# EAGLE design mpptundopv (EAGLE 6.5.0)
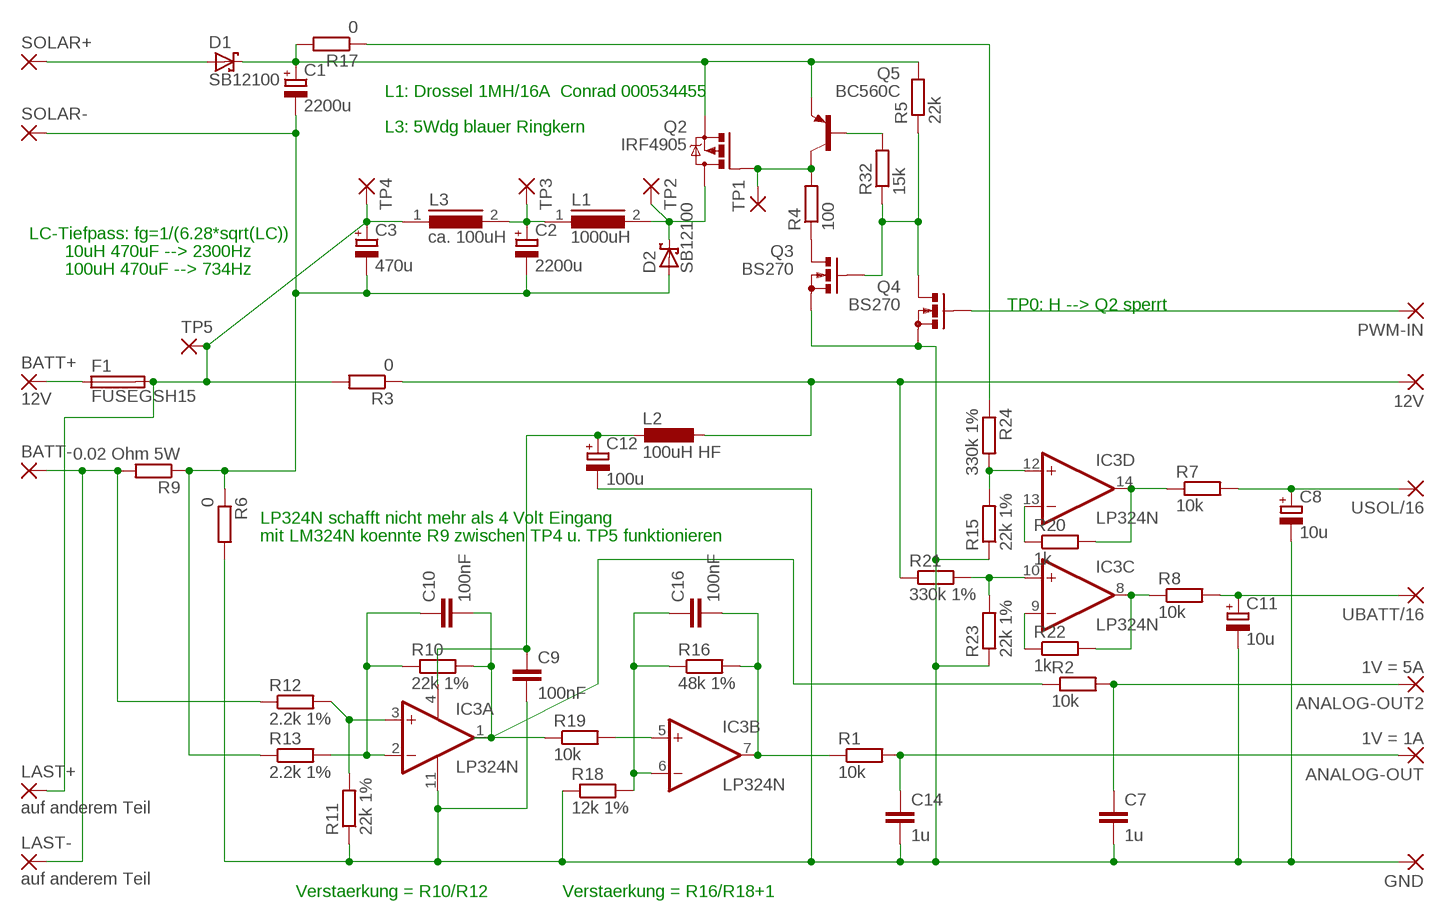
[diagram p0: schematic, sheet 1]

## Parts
12V  WIREPAD2,15/1,0  [2,15/1,0]
ANALOG-OUT  1V = 1A  WIREPAD2,15/1,0  [2,15/1,0]
ANALOG-OUT2  1V = 5A  WIREPAD2,15/1,0  [2,15/1,0]
BATT+  12V  WIREPAD3,81/1,1  [3,81/1,1]
BATT-  WIREPAD3,81/1,1  [3,81/1,1]
C1  2200u  CPOL-EUE7.5-18  [E7,5-18]
C2  2200u  CPOL-EUE7.5-18  [E7,5-18]
C3  470u  CPOL-EUE3.5-10  [E3,5-10]
C7  1u  C-EU025-025X050  [C025-025X050]
C8  10u  CPOL-EUE2.5-6  [E2,5-6]
C9  100nF  C-EUC1206  [C1206]
C10  100nF  C-EU025-024X044  [C025-024X044]
C11  10u  CPOL-EUE2.5-6  [E2,5-6]
C12  100u  CPOL-EUE5-13  [E5-13]
C14  1u  C-EU025-025X050  [C025-025X050]
C16  100nF  C-EU025-024X044  [C025-024X044]
D1  SB12100  1N5908  [C4111-15]
D2  SB12100  1N5908  [C4111-15]
F1  FUSEGSH15  [GSH15]
GND  WIREPAD2,15/1,0  [2,15/1,0]
IC3  LP324N  LM324N  [DIL14]
L1  1000uH  A26GFC  [A26GFC]
L2  100uH HF  L-EU0204/7  [0204/7]
L3  ca. 100uH  82114R  [82114R]
LAST+  auf anderem Teil  WIREPAD3,81/1,1  [3,81/1,1]
LAST-  auf anderem Teil  WIREPAD3,81/1,1  [3,81/1,1]
PWM-IN  WIREPAD2,15/1,0  [2,15/1,0]
Q2  IRF4905  IRF9530  [TO220BV]
Q3  BS270  BS170  [SOT54E]
Q4  BS270  BS170  [SOT54E]
Q5  BC560C  [TO92-EBC]
R1  10k  R-EU_0204/2V  [0204V@1]
R2  10k  R-EU_0204/2V  [0204V@1]
R3  0  R-EU_R1206  [R1206]
R4  100  R-EU_0204/5  [0204/5@1]
R5  22k  R-EU_0204/2V  [0204V@1]
R6  0  R-EU_R1206  [R1206]
R7  10k  R-EU_0204/5  [0204/5@1]
R8  10k  R-EU_0204/5  [0204/5@1]
R9  0.02 Ohm 5W  R-EU_0617/17  [0617/17]
R10  22k 1%  R-EU_0204/2V  [0204V@1]
R11  22k 1%  R-EU_0204/5  [0204/5@1]
R12  2.2k 1%  R-EU_0204/5  [0204/5@1]
R13  2.2k 1%  R-EU_0204/7  [0204/7@1]
R15  22k 1%  R-EU_0204/5  [0204/5@1]
R16  48k 1%  R-EU_0204/2V  [0204V@1]
R17  0  R-EU_R1206  [R1206]
R18  12k 1%  R-EU_0204/5  [0204/5@1]
R19  10k  R-EU_0207/10  [0207/10]
R20  1k  R-EU_0204/2V  [0204V@1]
R21  330k 1%  R-EU_0204/5  [0204/5@1]
R22  1k  R-EU_0204/2V  [0204V@1]
R23  22k 1%  R-EU_0204/2V  [0204V@1]
R24  330k 1%  R-EU_0204/7  [0204/7@1]
R32  15k  R-EU_0204/2V  [0204V@1]
SOLAR+  WIREPAD3,81/1,1  [3,81/1,1]
SOLAR-  WIREPAD3,81/1,1  [3,81/1,1]
TP1  WIREPAD2,15/1,0  [2,15/1,0]
TP2  WIREPAD3,17/1,2  [3,17/1,2]
TP3  WIREPAD3,17/1,2  [3,17/1,2]
TP4  WIREPAD3,17/1,2  [3,17/1,2]
TP5  WIREPAD3,17/1,2  [3,17/1,2]
UBATT/16  WIREPAD2,15/1,0  [2,15/1,0]
USOL/16  WIREPAD2,15/1,0  [2,15/1,0]

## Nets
GND [dick]: C7.2 C8.- C9.2 C11.- C12.- C14.2 GND.1(P) IC3.11(P:V-) Q3.S Q4.S R6.2 R11.1 R15.1 R18.1 R23.1
N$1 [dick]: ANALOG-OUT2.1(P) C7.1 R2.2
N$3 [duenn]: IC3.14(D:OUT) R7.1 R20.2
N$4 [duenn]: IC3.12(D:+IN) R15.2 R24.2
N$5 [sehrdick]: C1.- C2.- C3.- D2.A R6.1 R9.1 R13.1 SOLAR-.1(P)
N$6 [sehrdick]: D1.A SOLAR+.1(P)
N$7 [duenn]: PWM-IN.1(P) Q4.G
N$9 [sehrdick]: BATT+.1(P) F1.1
N$10 [duenn]: IC3.8(C:OUT) R8.1 R22.2
N$11 [dick]: C11.+ R8.2 UBATT/16.1(P)
N$12 [sehrdick]: C2.+ L1.1 L3.2 TP3.1(P)
N$13 [dick]: Q3.G Q4.D R5.1 R32.1
N$15 [dick]: Q3.D R4.1
N$16 [sehrdick]: C1.+ D1.C Q2.S Q5.E R5.2 R17.2
N$17 [sehrdick]: D2.C L1.2 Q2.D TP2.1(P)
N$19 [dick]: Q2.G Q5.C R4.2 TP1.1(P)
N$20 [duenn]: C16.2 IC3.7(B:OUT) R1.1 R16.2
N$21 [duenn]: C10.1 IC3.2(A:-IN) R10.1 R13.2
N$22 [dick]: C8.+ R7.2 USOL/16.1(P)
N$23: BATT-.1(P) LAST-.1(P) R9.2 R12.1
N$24 [duenn]: IC3.3(A:+IN) R11.2 R12.2
N$25 [duenn]: IC3.10(C:+IN) R21.2 R23.2
N$26 [duenn]: IC3.13(D:-IN) R20.1
N$27 [duenn]: IC3.9(C:-IN) R22.1
N$28 [duenn]: C16.1 IC3.6(B:-IN) R16.1 R18.2
N$29 [duenn]: IC3.5(B:+IN) R19.2
N$32 [sehrdick]: C3.+ F1.2 L3.1 LAST+.1(P) R3.2 TP4.1(P) TP5.1(P)
N$37 [duenn]: R17.1 R24.1
N$47 [duenn]: C10.2 IC3.1(A:OUT) R2.1 R10.2 R19.1
N$48 [dick]: Q5.B R32.2
N$51 [dick]: ANALOG-OUT.1(P) C14.1 R1.2
V12 [dick]: 12V.1(P) L2.1 R3.1 R21.1
V+ [dick]: C9.1 C12.+ IC3.4(P:V+) L2.2

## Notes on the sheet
- L1: Drossel 1MH/16A  Conrad 000534455
- L3: 5Wdg blauer Ringkern
- LC-Tiefpass: fg=1/(6.28*sqrt(LC))
- 10uH 470uF --> 2300Hz
- 100uH 470uF --> 734Hz
- TP0: H --> Q2 sperrt
- LP324N schafft nicht mehr als 4 Volt Eingang
- mit LM324N koennte R9 zwischen TP4 u. TP5 funktionieren
- Verstaerkung = R10/R12 | Verstaerkung = R16/R18+1

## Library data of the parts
12V ANALOG-OUT ANALOG-OUT2 BATT+ BATT- GND LAST+ LAST- PWM-IN SOLAR+ SOLAR- TP1-TP5 UBATT/16 USOL/16 = wirepad:WIREPAD: Wire PAD connect wire on PCB
C1-C3 C8 C11 C12 = rcl:CPOL-EU: POLARIZED CAPACITOR, European symbol
C7 C9 C10 C14 C16 = rcl:C-EU: CAPACITOR, European symbol
D1 D2 = diode:1N5908: DIODE
F1 = fuse:FUSE: Fuse; OC_FARNELL: unknown; OC_NEWARK: unknown
IC3 = linear:LM324: OP AMP
L1 = inductors:A26GFC: INDUCTOR
L2 = rcl:L-EU: INDUCTOR, European symbol
L3 = inductors:82114R: INDUCTOR
Q2 = transistor-power:IRF9530: P-CHANNEL HEXFET POWER-MOS-FET Source: http://www.irf.com/product-info/datasheets/data/irf9530.pdf
Q3 Q4 = transistor-small-signal:BS170: N-CHANNEL MOS FET
Q5 = transistor-pnp:BC560*: PNP Transistror
R1-R13 R15-R24 R32 = rcl:R-EU_: RESISTOR, European symbol

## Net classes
0 default: width 0.508 mm
1 dick: width 1.016 mm, clearance 0.203 mm
2 sehrdick: width 2.032 mm, clearance 0.508 mm
3 duenn: width 0.762 mm

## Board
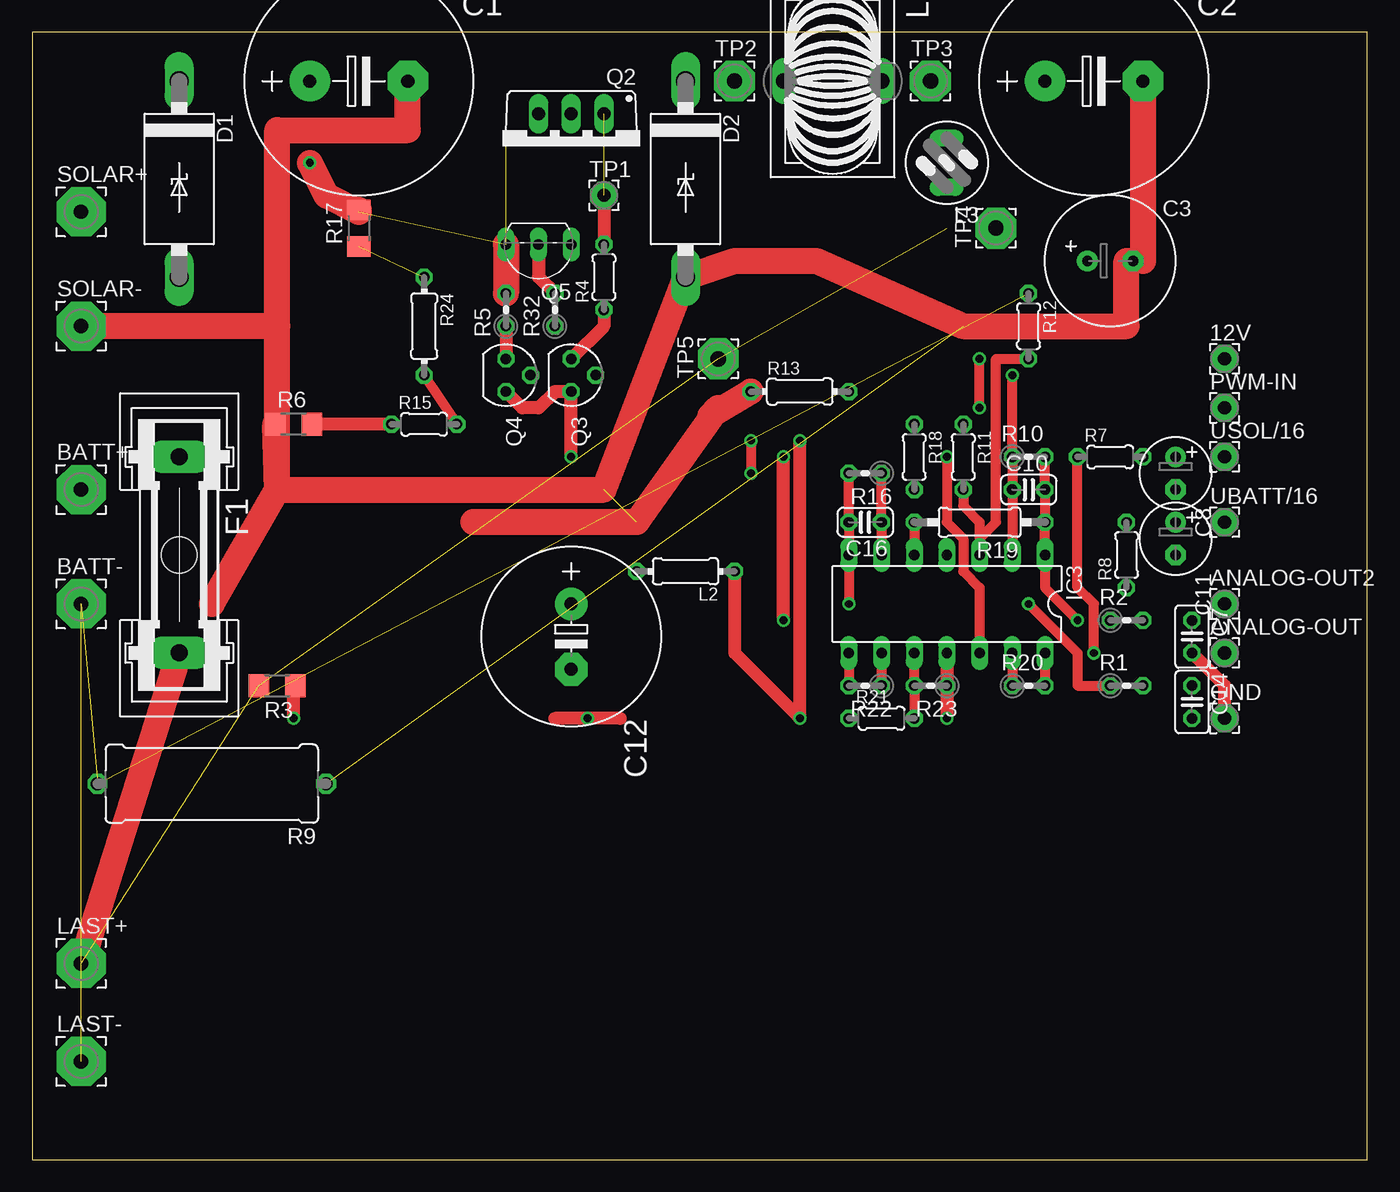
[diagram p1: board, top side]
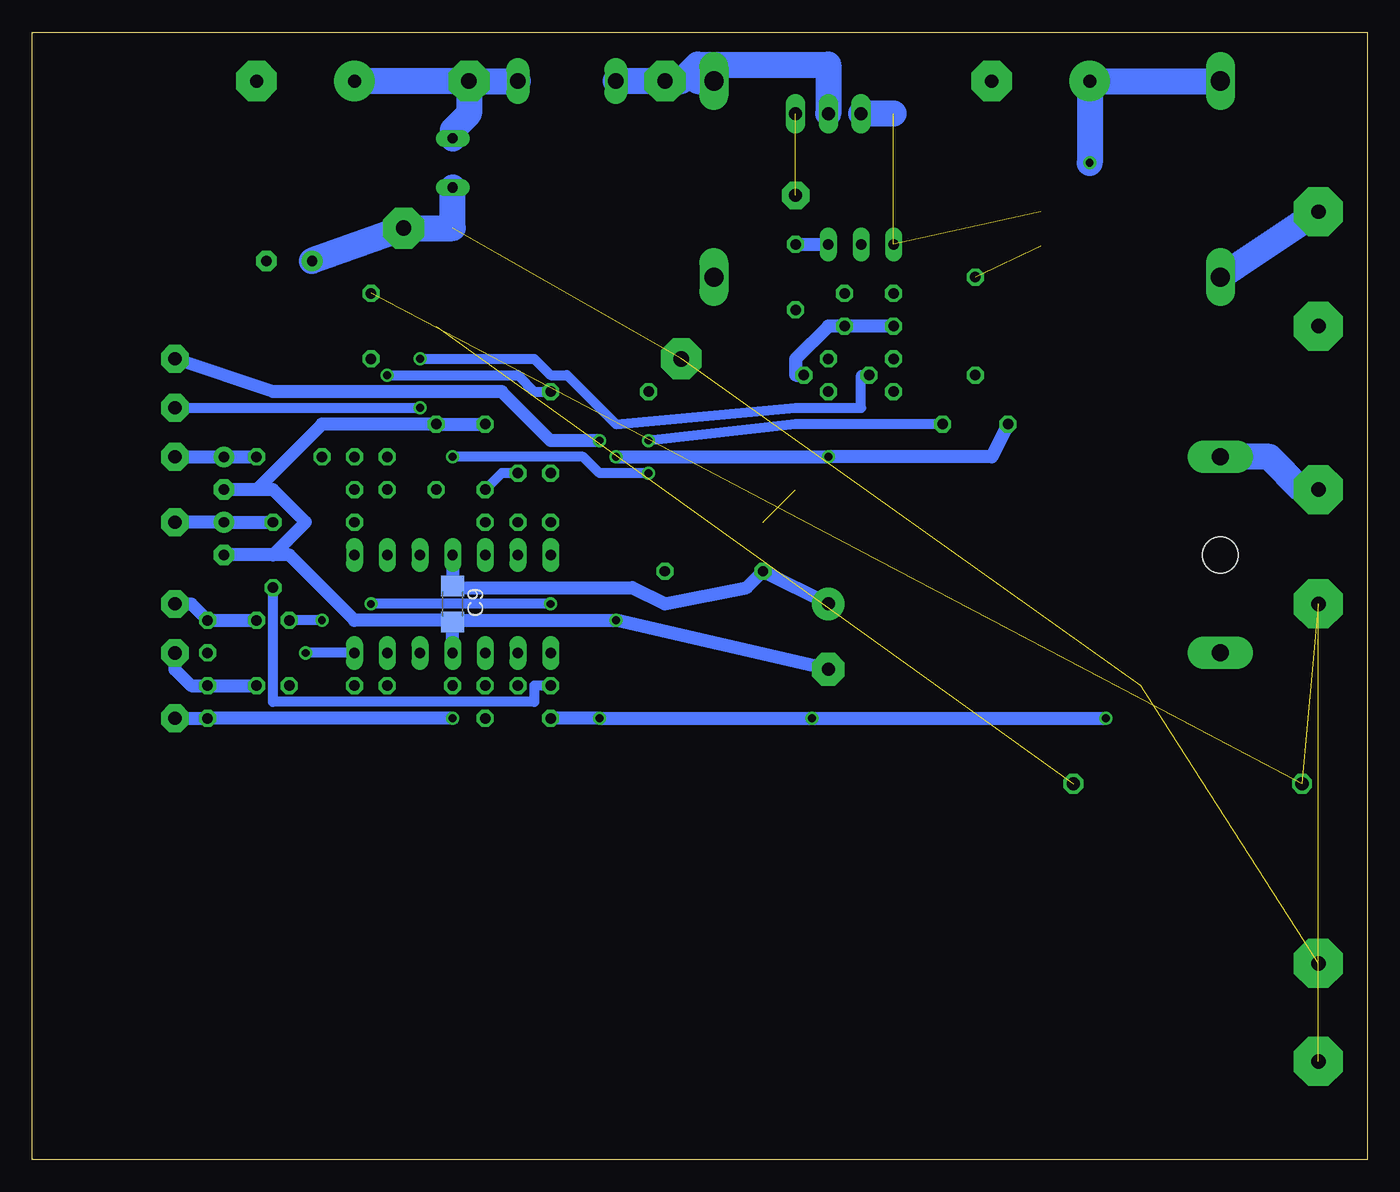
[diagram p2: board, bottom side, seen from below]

Size 103.81 x 87.62 mm. Coordinates in mm from the lower left corner, seen from the top.
Outline: 0,0 103.81,0 103.81,87.62 0,87.62 0,0
Copper layers (1*16): Top 0.035mm / dielectric 1.5mm / Bottom 0.035mm
Design rules "default": minimum track width 10mil, minimum drill 24mil, track to track 8mil, track to pad 8mil, pad to pad 8mil, via to via 8mil, smd to smd 8mil, copper to edge 40mil, drill to drill 8mil, minimum pad ring 10mil, minimum via ring 8mil, stop-mask expansion 4mil, vias tented up to drill 0mil, thermal gap 10mil

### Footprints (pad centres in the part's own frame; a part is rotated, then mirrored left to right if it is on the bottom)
2,15/1,0 = drill 1.016 pad 2.159 octagon: 1 0,0
3,81/1,1 = drill 1.118 pad 3.81 octagon: 1 0,0
E7,5-18 = drill 1.016 pad 3.15: + -3.81,0 | drill 1.016 pad 3.15 octagon: - 3.81,0
E3,5-10 = drill 0.813 pad 1.6: + -1.778,0 | drill 0.813 pad 1.6 octagon: - 1.778,0
C025-025X050 = drill 0.813 octagon: 1 -1.27,0; 2 1.27,0
E2,5-6 = drill 0.813 pad 1.6: + -1.27,0 | drill 0.813 pad 1.6 octagon: - 1.27,0
C1206 = smd 1.6 x 1.8: 1 -1.4,0; 2 1.4,0
C025-024X044 = drill 0.813 octagon: 1 -1.27,0; 2 1.27,0
E5-13 = drill 1.016 pad 2.54: + -2.54,0 | drill 1.016 pad 2.54 octagon: - 2.54,0
C4111-15 = drill 1.499 long: A 7.62,0; C -7.62,0
GSH15 = drill 1.321 pad 2.54 long: 1 -7.62,0; 2 7.62,0 | hole 2.794: 0,0
DIL14 = drill 0.813 long: 1 -7.62,-3.81; 2 -5.08,-3.81; 3 -2.54,-3.81; 4 0,-3.81; 5 2.54,-3.81; 6 5.08,-3.81; 7 7.62,-3.81; 8 7.62,3.81; 9 5.08,3.81; 10 2.54,3.81; 11 0,3.81; 12 -2.54,3.81; 13 -5.08,3.81; 14 -7.62,3.81
A26GFC = drill 1.194 long: 1 0,3.81; 2 0,-3.81
0204/7 = drill 0.813 octagon: 1 -3.81,0; 2 3.81,0
82114R = drill 0.813 long: 1 0,1.905; 2 0,-1.905
TO220BV = drill 1.016 long: D 0,-2.54; G -2.54,-2.54; S 2.54,-2.54
SOT54E = drill 0.813 octagon: D -1.27,0; G 0,1.905; S 1.27,0
TO92-EBC = drill 0.813 long: B 0,-1.27; C -2.54,-1.27; E 2.54,-1.27
0204V@1 = drill 0.813 octagon: 1 -1.27,0; 2 1.27,0
R1206 = smd 1.6 x 1.803: 1 -1.422,0; 2 1.422,0
0204/5@1 = drill 0.813 octagon: 1 -2.54,0; 2 2.54,0
0617/17 = drill 1.016 octagon: 1 -8.89,0; 2 8.89,0
0204/7@1 = drill 0.813 octagon: 1 -3.81,0; 2 3.81,0
0207/10 = drill 0.813 octagon: 1 -5.08,0; 2 5.08,0
3,17/1,2 = drill 1.194 pad 3.175 octagon: 1 0,0

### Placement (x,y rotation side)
12V  92.71,62.23 0 top
ANALOG-OUT  92.71,39.37 0 top
ANALOG-OUT2  92.71,43.18 0 top
BATT+  3.81,52.07 0 top
BATT-  3.81,43.18 0 top
C1  25.4,83.82 0 top
C2  82.55,83.82 0 top
C3  83.82,69.85 0 top
C7  90.17,40.64 270 top
C8  88.9,53.34 270 top
C9  71.12,43.18 270 bottom
C10  77.47,52.07 0 top
C11  88.9,48.26 270 top
C12  41.91,40.64 270 top
C14  90.17,35.56 270 top
C16  64.77,49.53 180 top
D1  11.43,76.2 270 top
D2  50.8,76.2 270 top
F1  11.43,46.99 270 top
GND  92.71,34.29 0 top
IC3  71.12,43.18 180 top
L1  62.23,83.82 270 top
L2  50.8,45.72 180 top
L3  71.12,77.47 180 top
LAST+  3.81,15.24 0 top
LAST-  3.81,7.62 0 top
PWM-IN  92.71,58.42 0 top
Q2  41.91,78.74 180 top
Q3  41.91,60.96 270 top
Q4  36.83,60.96 270 top
Q5  39.37,69.85 180 top
R1  85.09,36.83 0 top
R2  85.09,41.91 0 top
R3  19.05,36.83 180 top
R4  44.45,68.58 90 top
R5  36.83,66.04 90 top
R6  20.32,57.15 0 top
R7  83.82,54.61 0 top
R8  85.09,46.99 90 top
R9  13.97,29.21 180 top
R10  77.47,54.61 0 top
R11  72.39,54.61 270 top
R12  77.47,64.77 270 top
R13  59.69,59.69 0 top
R15  30.48,57.15 0 top
R16  64.77,53.34 180 top
R17  25.4,72.39 90 top
R18  68.58,54.61 270 top
R19  73.66,49.53 180 top
R20  77.47,36.83 0 top
R21  66.04,34.29 0 top
R22  64.77,36.83 180 top
R23  69.85,36.83 180 top
R24  30.48,64.77 270 top
R32  40.64,66.04 90 top
SOLAR+  3.81,73.66 0 top
SOLAR-  3.81,64.77 0 top
TP1  44.45,74.93 0 top
TP2  54.61,83.82 0 top
TP3  69.85,83.82 0 top
TP4  74.93,72.39 90 top
TP5  53.34,62.23 90 top
UBATT/16  92.71,49.53 0 top
USOL/16  92.71,54.61 0 top

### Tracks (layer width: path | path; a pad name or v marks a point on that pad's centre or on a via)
GND  (via drill 0.61)
  Top 1.016: R15.1 R6.2 | C7.2 92.71,36.83 GND.1 | IC3.11 R23.1 v71.12,34.29 | v58.42,41.91 v58.42,54.61 | v41.91,54.61 Q3.S 40.64,59.69 39.37,58.42 38.1,58.42 Q4.S
  Bottom 1.016: R15.1 29.21,54.61 v41.91,54.61 v58.42,54.61 | R18.1 R11.1 81.28,57.15 86.36,52.07 | 86.36,52.07 C8.- | GND.1 C14.2 v71.12,34.29 | IC3.11 C9.2 71.12,41.91 | 85.09,46.99 83.82,46.99 78.74,41.91 71.12,41.91 | 85.09,46.99 C11.- | 86.36,52.07 85.09,52.07 82.55,49.53 85.09,46.99 | 71.12,41.91 v58.42,41.91 C12.-
N$1
  Bottom 1.016: R2.2 C7.1 91.44,43.18 ANALOG-OUT2.1
N$3  (via drill 0.61)
  Top 0.762: IC3.14 R20.2 | R7.1 81.28,44.45 82.55,43.18 v82.55,39.37
  Bottom 0.762: IC3.14 v82.55,39.37
N$4  (via drill 0.61)
  Top 0.762: R24.2 R15.2 | IC3.12 73.66,44.45 72.39,45.72 72.39,48.26 71.12,49.53 v71.12,54.61 | v55.88,55.88 v55.88,53.34
  Bottom 0.762: v71.12,54.61 60.96,54.61 59.69,53.34 v55.88,53.34 | R15.2 44.45,57.15 v55.88,55.88
N$5  (2 unrouted)
  Top 2.032: R13.1 52.7,57.78 53.34,58.42 46.99,49.53 34.29,49.53 | C2.- 86.36,69.85 C3.- 85.09,69.85 85.09,64.77 72.39,64.77 60.96,69.85 54.61,69.85 D2.A 44.45,52.07 19.05,52.07 | 13.97,43.18 19.05,52.07 | 19.05,52.07 R6.1 | C1.- 29.21,80.01 19.05,80.01 19.05,64.77 | 19.05,52.07 19.05,64.77 | 19.05,64.77 SOLAR-.1
N$6
  Bottom 2.032: SOLAR+.1 D1.A
N$7  (via drill 0.61)
  Top 0.762: v73.66,58.42 v73.66,62.23
  Bottom 0.762: v73.66,62.23 64.77,62.23 63.5,60.96 62.23,60.96 58.42,57.15 44.45,58.42 39.37,58.42 39.37,60.96 Q4.G | PWM-IN.1 v73.66,58.42
N$9
  Bottom 2.032: F1.1 7.62,54.61 5.08,52.07 BATT+.1
N$10
  Top 0.762: IC3.8 R22.2
  Bottom 0.762: R8.1 85.09,35.56 64.77,35.56 64.77,36.83 R22.2
N$11
  Bottom 1.016: R8.2 C11.+ UBATT/16.1
N$12
  Bottom 2.032: TP3.1 69.85,81.28 71.12,80.01 L3.2 | TP3.1 L1.1 | TP3.1 C2.+
N$13
  Top 1.016: R5.1 Q4.D
  Bottom 1.016: R5.1 R32.1 41.91,64.77 44.45,62.23 44.45,60.96 Q3.G
N$15
  Top 1.016: Q3.D 44.45,64.77 R4.1
N$16  (via drill 0.61)  (2 unrouted)
  Top 2.032: Q5.E R5.2 | v21.59,77.47 22.86,74.93 25.4,73.66 R17.2
  Bottom 2.032: 36.83,81.28 Q2.S | v21.59,77.47 C1.+ D1.C
N$17
  Bottom 2.032: Q2.D 41.91,85.09 52.07,85.09 52.7,84.46 | 52.7,84.46 53.34,83.82 TP2.1 L1.2 | D2.C 52.07,83.82 52.7,84.46
N$19  (1 unrouted)
  Top 1.016: TP1.1 R4.2
  Bottom 1.016: R4.2 Q5.C
N$20  (via drill 0.61)
  Top 0.762: R16.2 C16.2 IC3.7 v63.5,43.18 | R1.1 81.28,36.83 81.28,39.37 v77.47,43.18
  Bottom 0.762: v63.5,43.18 v77.47,43.18
N$21  (via drill 0.61)
  Top 0.762: IC3.2 C10.1 R10.1 v76.2,60.96
  Bottom 0.762: R13.2 64.77,59.69 66.04,60.96 v76.2,60.96
N$22
  Bottom 1.016: R7.2 C8.+ USOL/16.1
N$23  (3 unrouted)
N$24
  Top 0.762: 73.66,48.26 73.66,49.53 72.39,50.8 R11.2 | R12.2 74.93,62.23 74.93,49.53 73.66,48.26 | 73.66,48.26 IC3.3
N$25
  Top 0.762: R21.2 R23.2 IC3.10
N$26
  Top 0.762: IC3.13 R20.1
N$27
  Top 0.762: IC3.9 R22.1
N$28
  Top 0.762: IC3.6 C16.1 R16.1
  Bottom 0.762: R18.2 67.31,53.34 R16.1
N$29
  Top 0.762: R19.2 IC3.5
N$32  (3 unrouted)
  Top 2.032: F1.2 LAST+.1
  Bottom 2.032: L3.1 71.12,72.39 TP4.1 C3.+
N$37  (1 unrouted)
  Top 0.762: 25.4,71.12 R17.1
N$47  (via drill 0.61)
  Top 0.762: R10.2 C10.2 R19.1 IC3.1 78.74,44.45 v81.28,41.91
  Bottom 0.762: v81.28,41.91 R2.1
N$48
  Top 1.016: R32.2 39.37,68.58 Q5.B
N$51
  Bottom 1.016: R1.2 C14.1 91.44,36.83 92.71,38.1 ANALOG-OUT.1
V12  (via drill 0.61)
  Top 1.016: 45.72,34.29 v43.18,34.29 40.64,34.29 | v20.32,34.29 20.32,36.83 R3.1 | v59.69,55.88 v59.69,34.29 54.61,39.37 L2.1
  Bottom 1.016: v20.32,34.29 v43.18,34.29 v59.69,34.29 R21.1 | 12V.1 85.09,59.69 67.31,59.69 63.5,55.88 v59.69,55.88
V+
  Bottom 1.016: IC3.4 C9.1 71.12,44.45 57.15,44.45 54.61,43.18 48.26,44.45 L2.2 C12.+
